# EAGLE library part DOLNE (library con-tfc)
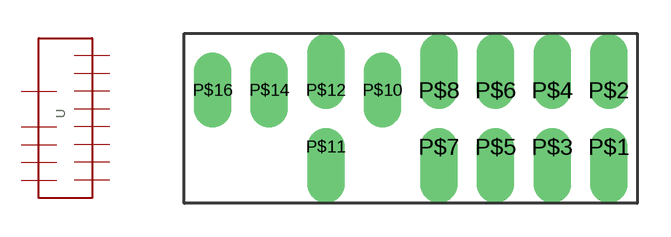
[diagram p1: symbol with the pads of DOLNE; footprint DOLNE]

Designator prefix -

## DOLNE  [DOLNE]
P$1  P$1  pas
P$2  P$2  pas
P$3  P$3  pas
P$4  P$4  pas
P$5  P$5  pas
P$6  P$6  pas
P$7  P$7  pas
P$8  P$8  pas
P$10  P$10  pas
P$11  P$11  pas
P$12  P$12  pas
P$14  P$14  pas
P$16  P$16  pas

## Footprint DOLNE (pad centres in mm)
drill 0.5 pad 1.676 offset: P$1 8.89,-1.27; P$2 8.89,1.27; P$3 6.35,-1.27; P$4 6.35,1.27; P$5 3.81,-1.27; P$6 3.81,1.27; P$7 1.27,-1.27; P$8 1.27,1.27; P$11 -3.81,-1.27; P$12 -3.81,1.27
drill 0.5 pad 1.676 long: P$10 -1.27,1.27; P$14 -6.35,1.27; P$16 -8.89,1.27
